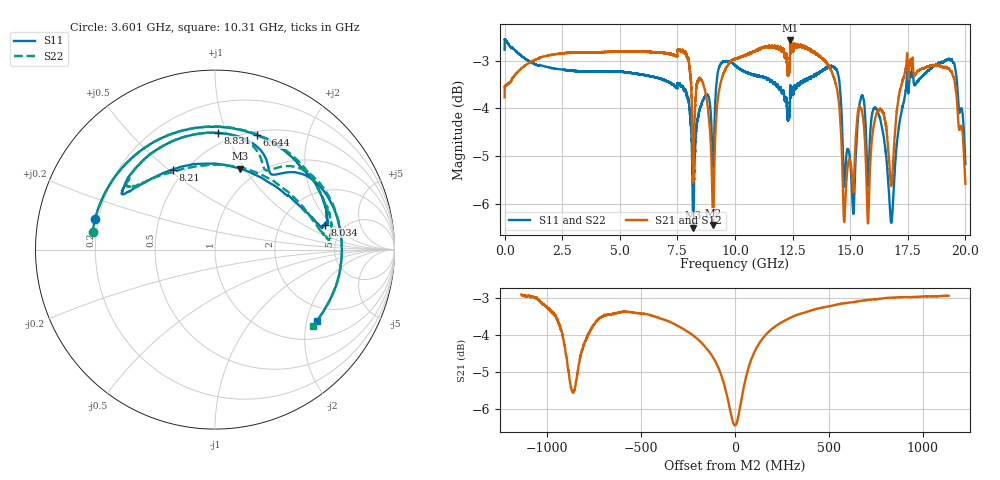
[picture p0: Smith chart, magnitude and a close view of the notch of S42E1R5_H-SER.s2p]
!{S42E1R5}
!Johanson Technology Inc.
!www.johansontechnology.com
!Test Board Conditions:
!Substrate Type  RO4350B
!Substrate Thickness  50 mil
!Substrate Dk  3.66
!TL Type: GCPW
!TL Trace Width  60 mil
!TL Gap  10 mil
!Electrode orientation  Horizontal
!DUT TOPOLOGY	SERIES
!Mounting Pad LxW  14x55 mil
! Created Wed Nov 25 21:34:25 2020
# khz S ma R 50
! 2 Port Network Data from SP1.SP block
! freq  magS11  angS11  magS21  angS21  magS12  angS12  magS22  angS22
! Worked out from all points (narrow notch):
!   20001 points, 300 kHz to 20 GHz, reference 50 ohm
!   highest |S21| = -2.57 dB at 12.4 GHz (marker M1); lowest = -6.4 dB at 9.051 GHz (marker M2)
!   notch at M2: 3.5 dB deep, 190 MHz wide at half that depth
!   lowest |S11| = -6.5 dB at 8.187 GHz (marker M3), VSWR 2.79, Z = 41.2 + j47.9 ohm
!   |S11| at or under -10 dB: nowhere
!   |S22| runs from -6.5 to -2.5 dB; largest |S21 - S12| = 0.12
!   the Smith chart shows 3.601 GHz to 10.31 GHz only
!   S11 on the Smith chart (normalised r, x): 3.601 GHz: 0.19, +0.12; 6.644 GHz: 0.54, +1.29; 8.034 GHz: 3.56, +1.64; 8.21 GHz: 0.44, +0.52; 8.831 GHz: 0.42, +0.94; 10.31 GHz: 1.50, -2.29
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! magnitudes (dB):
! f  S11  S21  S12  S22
! 300 kHz  -2.8  -3.8  -3.8  -2.8
! 3.334 GHz  -3.2  -2.8  -2.8  -3.2
! 3.601 GHz  -3.2  -2.8  -2.8  -3.2
! 6.644 GHz  -3.4  -2.8  -2.8  -3.4
! 6.667 GHz  -3.4  -2.8  -2.8  -3.4
! 8.034 GHz  -4.0  -3.2  -3.2  -4.1
! 8.187 GHz  -6.5  -5.6  -5.6  -6.5
! 8.21 GHz  -6.0  -5.0  -5.0  -6.0
! 8.831 GHz  -3.7  -4.0  -4.0  -3.7
! 9.051 GHz  -5.6  -6.4  -6.4  -5.6
! 10 GHz  -3.1  -3.0  -3.0  -3.1
! 10.31 GHz  -3.2  -2.9  -2.9  -3.2
! 12.4 GHz  -3.5  -2.6  -2.6  -3.5
! 13.33 GHz  -3.3  -2.8  -2.8  -3.3
! 14.42 GHz  -3.2  -3.6  -3.6  -3.2
! 14.76 GHz  -5.6  -6.3  -6.3  -5.6
! 15.52 GHz  -3.7  -4.1  -4.1  -3.7
! 15.77 GHz  -5.7  -6.4  -6.4  -5.6
! 16.2 GHz  -4.1  -4.1  -4.1  -4.1
! 16.67 GHz  -5.7  -5.0  -5.0  -5.7
! 18.9 GHz  -3.1  -3.1  -3.1  -3.1
! 20 GHz  -5.2  -5.6  -5.6  -5.3
